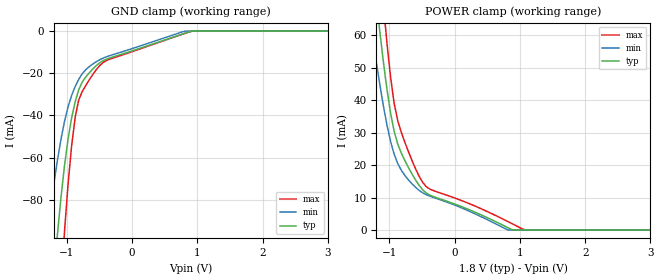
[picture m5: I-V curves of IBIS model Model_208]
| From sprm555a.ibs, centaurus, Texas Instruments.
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| Model based on original model for BCSHTLTCSCDVPBFZ_SSGFV
|   Sub model VREF_HALFTERM_8MA_10PER_1P8
[model]   Model_208
|[Description]  [1.8V-INPUT-HALFTERM:8MA-X, IND, 10%]
|   Half Thevenin termination (Rth = 100R whith RExt = 50R)
|   (ODT[1:0] = "11") VRef mode, 1.00 * RExt = 1.000 * Iout (I[2:0]
|   = "011"), 8mA nominal with Rext = 50R,Industrial temperature
|   range (-40C to 125C, 25C nominal),10% power supply tolerance
|[Input Load]   HALFTERM:8MA
|[Output Drive]
|Voltage   1.8V
|Mode   INPUT
Model_type   Input
Polarity   Non-Inverting
Vinl =  0.775
Vinh =  1.025
C_comp   1.851324p   1.663768p   1.973575p
[Model Spec]
Vinl   0.775   0.685   0.865
Vinh   1.025   0.935   1.115
[Temperature Range]   25   125   -40
[Voltage Range]   1.8   1.62   1.98
[POWER_clamp]
-1.8V     200.5mA    141mA      270.2mA
-1.309V   92.78mA    66.7mA     123.5mA
-1.255V   81.7mA     59.09mA    109mA
-1.145V   60.96mA    44.71mA    81.81mA
-1.091V   51.63mA    38.16mA    69.19mA
-1.036V   43.24mA    32.27mA    57.48mA
-927.3mV  30.46mA    23.36mA    39.05mA
-872.7mV  26.55mA    20.51mA    33.74mA
-490.9mV  12.43mA    11.47mA    14.71mA
818.2mV   689.3uA    0A         2.566mA
1.091V    0A         0A         0A
3.6V      0A         0A         0A
[GND_clamp]
-1.8V     -356.1mA   -217.5mA   -579.1mA
-1.309V   -156.2mA   -96.5mA    -253mA
-1.145V   -96.65mA   -61.37mA   -152.3mA
-1.036V   -63.77mA   -42.84mA   -95.02mA
-927.3mV  -41.19mA   -30.5mA    -54.42mA
-872.7mV  -33.5mA    -26.25mA   -40.88mA
-818.2mV  -27.78mA   -22.84mA   -32.58mA
-763.6mV  -24.12mA   -20.19mA   -28.62mA
-545.5mV  -16.23mA   -14.44mA   -18.11mA
-381.8mV  -13.17mA   -12.06mA   -13.8mA
927.3mV   0A         0A         0A
3.6V      0A         0A         0A
